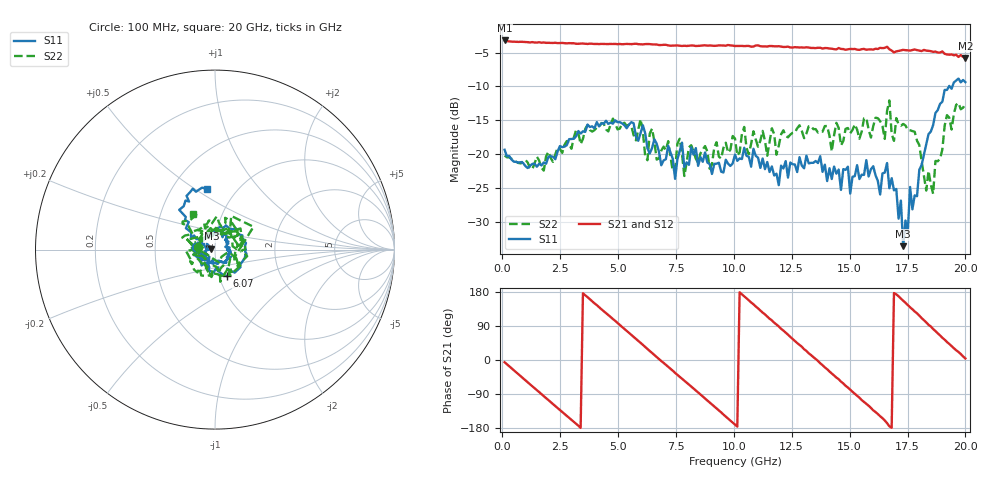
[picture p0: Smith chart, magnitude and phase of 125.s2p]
!Agilent Technologies,N5230C,MY49001569,A.09.33.09
!Agilent N5230C: A.09.33.09
!Date: Monday, July 20, 2015 20:31:40
!Correction: S11(Full 2 Port(1,2))
!S21(Full 2 Port(1,2))
!S12(Full 2 Port(1,2))
!S22(Full 2 Port(1,2))
!S2P File: Measurements: S11, S21, S12, S22:
# Hz S  dB  R 50
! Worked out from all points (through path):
!   201 points, 100 MHz to 20 GHz, reference 50 ohm
!   highest |S21| = -3.21 dB at 100 MHz (marker M1); lowest = -5.8 dB at 20 GHz (marker M2)
!   group delay of S21, straight-line fit = 149 ps
!   lowest |S11| = -33.6 dB at 17.31 GHz (marker M3), VSWR 1.04, Z = 48 + j0.445 ohm
!   |S11| at or under -10 dB: start of sweep to 19.29 GHz; 19.32 GHz to 19.44 GHz (118 MHz wide, 0.609 % of centre)
!   |S22| runs from -25.9 to -12.1 dB; largest |S21 - S12| = 0.018
!   S11 on the Smith chart (normalised r, x): 100 MHz: 0.81, +0.03; 6.07 GHz: 1.09, -0.33; 20 GHz: 0.74, +0.56
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1e8  -19.35 170.9  -3.21 -6.0  -3.16 -5.6  -20.20 173.0
1.692e9  -21.67 115.1  -3.55 -90.1  -3.50 -89.9  -22.02 104.3
3.483e9  -16.62 52.0  -3.66 176.0  -3.66 175.9  -17.74 45.6
4.876e9  -15.00 -7.7  -3.72 103.3  -3.70 103.1  -15.42 -19.2
6.07e9  -15.73 -65.7  -3.80 40.0  -3.79 40.2  -16.62 -78.9
6.7665e9  -19.66 -107.6  -3.89 2.6  -3.88 2.9  -20.64 -133.4
8.5575e9  -20.43 175.6  -3.99 -91.0  -3.94 -91.0  -19.89 153.4
1.005e10  -20.06 91.5  -4.03 -170.4  -3.97 -170.0  -17.69 54.6
1.17415e10  -23.15 21.9  -4.08 98.5  -4.05 99.6  -17.04 -55.5
1.3433e10  -21.28 -52.3  -4.32 7.6  -4.42 7.2  -16.31 -145.5
1.5224e10  -23.24 -117.7  -4.46 -89.2  -4.53 -88.1  -15.61 100.9
1.65175e10  -22.72 -164.6  -4.31 -159.6  -4.24 -159.4  -17.75 50.1
1.67165e10  -25.04 -161.6  -4.51 -175.1  -4.35 -173.6  -12.07 30.6
1.69155e10  -25.34 -157.6  -4.99 176.6  -5.03 176.9  -18.03 52.7
1.7214e10  -26.85 178.1  -4.68 162.0  -4.66 162.7  -15.81 26.5
1.73135e10  -33.59 167.2  -4.60 156.7  -4.63 157.3  -15.54 25.8
1.75125e10  -31.48 156.5  -4.68 144.9  -4.60 145.3  -16.41 12.6
1.7612e10  -24.85 143.6  -4.71 139.1  -4.55 139.9  -16.48 9.3
1.77115e10  -28.14 159.4  -4.63 133.8  -4.65 134.5  -16.59 13.4
1.8607e10  -15.71 144.0  -4.90 81.7  -4.76 82.4  -25.86 -145.2
1.9204e10  -10.52 125.8  -5.28 47.5  -5.20 49.0  -14.24 159.8
2e10  -9.36 97.3  -5.79 4.0  -5.57 4.5  -12.59 121.5
